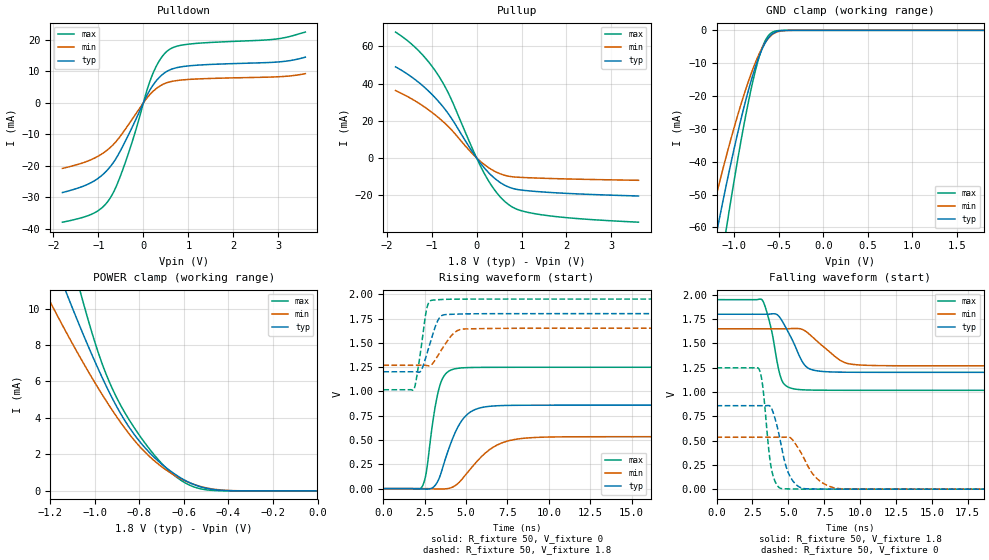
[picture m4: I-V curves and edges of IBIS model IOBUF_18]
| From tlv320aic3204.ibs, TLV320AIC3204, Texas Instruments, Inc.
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[Model]   IOBUF_18
Model_type  I/O
Vinl=0.495
Vinh=1.365
Enable   Active-Low
Vref =   0
|Rref =   50
Cref =   10p
Vmeas =   0.9
| variable   typ   min   max
C_comp   1.70pF   1.60pF   1.79pF
| C_pullup   3.53pF   1.82pF   4.67pF
| C_pulldown   2.75pF   1.81pF   3.50pF
| C_tri-state   1.70pF   1.60pF   1.79pF
[Temperature Range]   40   100   -40
| Ambient temperature   25   85   -40
[Voltage range]   1.8   1.65   1.95
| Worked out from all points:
|   slope of the pulldown table from 0 to 0.27 V, typ, clamps not added: 40.3 ohm
|   slope of the pullup table from 0 to 0.27 V, typ, clamps not added: 33.7 ohm
|   GND clamp passes 1 mA (typ) near -0.57 V on its own axis
|   POWER clamp passes 1 mA (typ) near -0.65 V on its own axis
|   rising waveform, R_fixture 50, V_fixture 0: 20-80 % time 1.18ns typ, 1.85ns min, 653ps max; typ from 0 V to 0.859 V
|   falling waveform, R_fixture 50, V_fixture 1.8: 20-80 % time 1.18ns typ, 1.8ns min, 758ps max; typ from 1.8 V to 1.2 V
|   rising waveform, R_fixture 50, V_fixture 1.8: 20-80 % time 651ps typ, 902ps min, 462ps max; typ from 1.2 V to 1.8 V
|   falling waveform, R_fixture 50, V_fixture 0: 20-80 % time 843ps typ, 1.35ns min, 510ps max; typ from 0.859 V to 0 V
[GND Clamp]
| IOBUF_18
|   Voltage   I(typ)   I(min)   I(max)
-1.8V     -152.2mA   -121.7mA   -195.2mA
-1.29V    -74.34mA   -59.83mA   -96.33mA
-1.18V    -58.98mA   -47.7mA    -76.25mA
-1.08V    -45.72mA   -37.25mA   -58.7mA
-910mV    -25.36mA   -21.17mA   -31.36mA
-785mV    -12.96mA   -11.28mA   -14.69mA
-730mV    -8.528mA   -7.687mA   -8.884mA
-675mV    -4.944mA   -4.718mA   -4.448mA
-625mV    -2.58mA    -2.675mA   -1.868mA
-575mV    -1.115mA   -1.308mA   -599uA
-390mV    -11.92uA   -29.16uA   -1.238uA
1.8V      55.79pA    47.12nA    25.49pA
[POWER Clamp]
| IOBUF_18
|   Voltage   I(typ)   I(min)   I(max)
-1.8V     35.6mA     26.77mA    51.61mA
-1.21V    13.49mA    10.59mA    17.9mA
-1.12V    10.62mA    8.51mA     13.45mA
-1.06V    8.814mA    7.194mA    10.68mA
-970mV    6.299mA    5.345mA    7.071mA
-890mV    4.366mA    3.858mA    4.833mA
-780mV    2.442mA    2.195mA    2.711mA
-705mV    1.529mA    1.376mA    1.578mA
-640mV    915.8uA    840.9uA    822.1uA
-555mV    351.9uA    358uA      219.9uA
-460mV    65.25uA    85.92uA    20.09uA
-16.28fV  55.79pA    535.9pA    32.67pA
[Pulldown]
| IOBUF_18
|   Voltage   I(typ)   I(min)   I(max)
-1.8V     -28.51mA   -20.84mA   -37.93mA
-1.095V   -24.82mA   -17.63mA   -35.02mA
-890mV    -22.63mA   -15.93mA   -32.94mA
-725mV    -20.08mA   -14.05mA   -29.96mA
-570mV    -16.76mA   -11.65mA   -25.4mA
-355mV    -10.87mA   -7.421mA   -17.02mA
180mV     4.875mA    3.155mA    8.179mA
355mV     8.092mA    5.218mA    13.38mA
545mV     10.16mA    6.486mA    16.61mA
950mV     11.64mA    7.364mA    18.54mA
2.885V    12.87mA    8.204mA    20.15mA
3.6V      14.5mA     9.265mA    22.47mA
[Pullup]
| IOBUF_18
|   Voltage   I(typ)   I(min)   I(max)
-1.8V     48.97mA    36.19mA    67.68mA
-1.285V   40.59mA    29.44mA    57.59mA
-1.06V    35.78mA    25.71mA    51.46mA
-855mV    30.61mA    21.82mA    44.59mA
-585mV    22.28mA    15.77mA    32.76mA
-105mV    3.734mA    2.563mA    5.689mA
165mV     -5.198mA   -3.48mA    -8.078mA
425mV     -11.49mA   -7.509mA   -18.04mA
690mV     -15.49mA   -9.784mA   -24.75mA
970mV     -17.27mA   -10.52mA   -28.29mA
1.49V     -18.42mA   -11.02mA   -30.82mA
3.6V      -20.56mA   -12.1mA    -34.65mA
[Ramp]
| IOBUF_18
| variable   typ   min   max
dV/dt_r   0.52/1.19E-09   0.32/1.86E-09   0.75/6.57E-10
dV/dt_f   0.36/1.19E-09   0.23/1.81E-09   0.56/7.67E-10
R_load = 50
[Rising Waveform]
| IOBUF_18
R_fixture =   50
C_fixture =   0
L_fixture =   0
V_fixture =   0
V_fixture_min = 0
V_fixture_max = 0
|   Time   V(typ)   V(min)   V(max)
0s        1.726nV    16.57nV    574pV
2.33ns    -3.51mV    -25.45uV   18.01mV
2.58ns    -4.93mV    310.4uV    155.4mV
3.06ns    21.08mV    -3.022mV   770mV
3.425ns   131mV      -3.838mV   1.067V
4.6ns     663.7mV    67.99mV    1.24V
5.41ns    803.2mV    232.5mV    1.246V
6.715ns   850.9mV    433.9mV    1.248V
9.29ns    858.2mV    527.2mV    1.248V
70ns      858.8mV    534.2mV    1.248V
[Falling Waveform]
| IOBUF_18
R_fixture =   50
C_fixture =   0
L_fixture =   0
V_fixture =   1.8
V_fixture_min = 1.65
V_fixture_max = 1.95
|   Time   V(typ)   V(min)   V(max)
0s        1.8V       1.65V      1.95V
3.17ns    1.8V       1.65V      1.949V
3.75ns    1.802V     1.65V      1.687V
4.295ns   1.787V     1.65V      1.255V
4.54ns    1.738V     1.65V      1.123V
5.74ns    1.381V     1.652V     1.025V
6.715ns   1.226V     1.562V     1.019V
8.73ns    1.204V     1.316V     1.018V
10.38ns   1.202V     1.275V     1.017V
70ns      1.202V     1.269V     1.017V
[Rising Waveform]
| IOBUF_18
R_fixture =   50
C_fixture =   0
L_fixture =   0
V_fixture =   1.8
V_fixture_min = 1.65
V_fixture_max = 1.95
|   Time   V(typ)   V(min)   V(max)
0s        1.202V     1.269V     1.017V
1.835ns   1.202V     1.269V     1.018V
2.255ns   1.208V     1.269V     1.42V
2.625ns   1.385V     1.267V     1.855V
2.8ns     1.483V     1.264V     1.928V
3.155ns   1.677V     1.33V      1.942V
3.515ns   1.779V     1.429V     1.945V
4.175ns   1.794V     1.585V     1.949V
5.025ns   1.798V     1.643V     1.95V
70ns      1.8V       1.65V      1.95V
[Falling Waveform]
| IOBUF_18
R_fixture =   50
C_fixture =   0
L_fixture =   0
V_fixture =   0
V_fixture_min = 0
V_fixture_max = 0
|   Time   V(typ)   V(min)   V(max)
0s        858.8mV    534.2mV    1.248V
2.955ns   858.8mV    534.2mV    1.237V
3.22ns    858.7mV    534.2mV    1.058V
3.82ns    835.2mV    534.2mV    213mV
4.545ns   423.2mV    534mV      5.4mV
5.01ns    166.5mV    536.8mV    2.559mV
5.69ns    29.69mV    422.5mV    1.066mV
6.995ns   1.706mV    109.8mV    328.4uV
8.7ns     392.8uV    3.78mV     96.88uV
70ns      84.02nV    91.36nV    80.56nV
